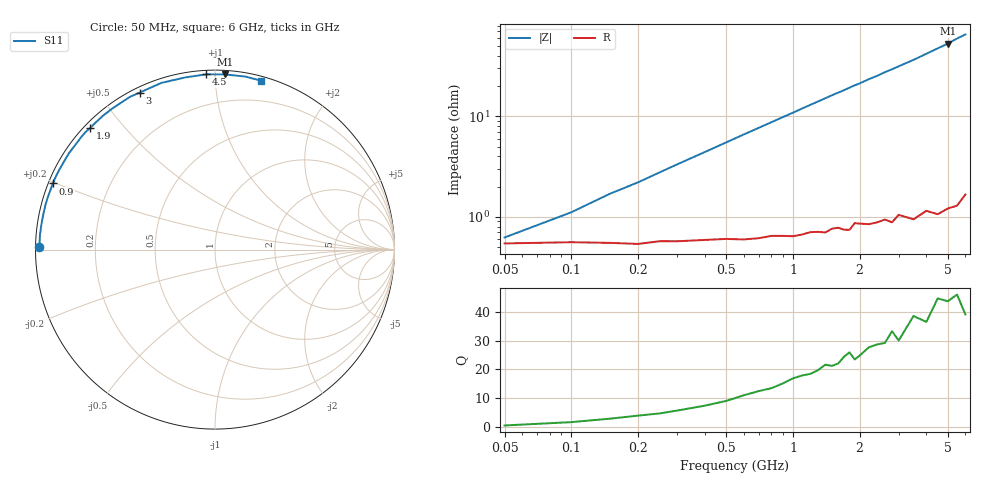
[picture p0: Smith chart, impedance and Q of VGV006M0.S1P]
! Infineon Technologies  Discrete & RF Semiconductors
! BB 831
! Si Tuning Diode in SOD323
! VR =
! S-Parameters:  July  1999
# GHz  S  MA  R  50
!  f  S11
! GHz  MAG  ANG
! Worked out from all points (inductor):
!   34 points, 50 MHz to 6 GHz, reference 50 ohm
!   read as one part to ground: L = 1.72 nH near 200 MHz
!   highest Q = 44.6 at 5 GHz (marker M1), where L = 1.69 nH
!   S11 on the Smith chart (normalised r, x): 50 MHz: 0.01, +0.01; 900 MHz: 0.01, +0.20; 1.9 GHz: 0.02, +0.41; 3 GHz: 0.02, +0.63; 4.5 GHz: 0.02, +0.95; 6 GHz: 0.03, +1.31
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0.05  0.9785 179.3
0.15  0.9782 176.3
0.2  0.9787 175.1
0.4  0.9769 170.0
0.6  0.9768 165.0
0.7  0.9763 162.6
0.8  0.9752 160.2
0.9  0.9754 157.8
1  0.9758 155.5
1.1  0.975 153.1
1.2  0.9739 150.8
1.4  0.9747 146.3
1.6  0.9725 142.0
1.7  0.974 140.0
1.8  0.9744 137.8
1.9  0.9707 135.7
2  0.9714 133.9
2.2  0.9726 129.8
2.4  0.9723 126.3
2.6  0.9715 122.4
2.8  0.9741 119.1
3  0.9704 115.6
3.5  0.9756 107.8
4  0.9734 100.0
4.5  0.9779 93.0
5  0.9774 86.7
5.5  0.9788 80.1
6  0.9756 74.9
